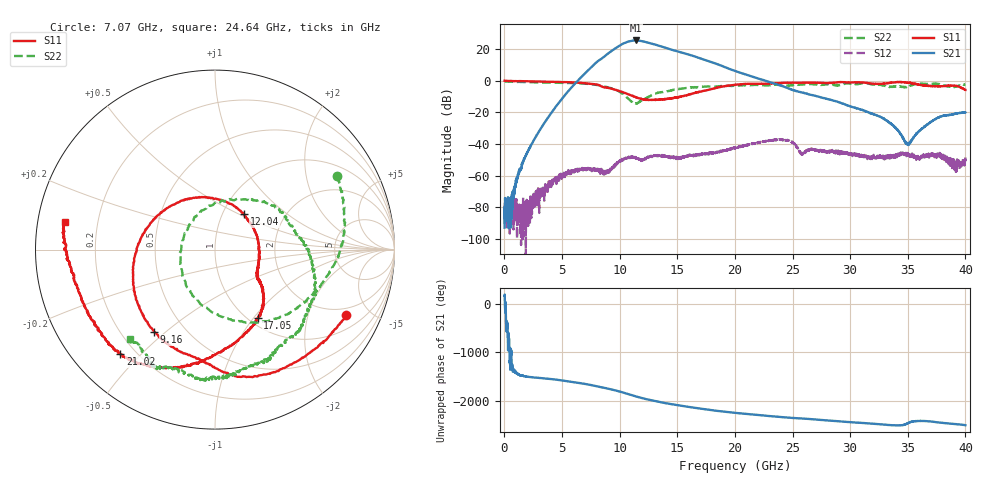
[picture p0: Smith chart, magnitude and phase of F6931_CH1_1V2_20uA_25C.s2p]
!Keysight Technologies,M9807A,MY58100526,A.15.20.05
!Date: Wednesday, October 25, 2023 15:38:21
!Correction: S11(C  2-Port  )
!S21(C  2-Port  )
!S12(C  2-Port  )
!S22(C  2-Port  )
!S2P File: Measurements: S11, S21, S12, S22:
# Hz S  dB  R 50
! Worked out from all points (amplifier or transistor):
!   4000 points, 10 MHz to 40 GHz, reference 50 ohm
!   highest |S21| = 25.3 dB at 11.4 GHz (marker M1)
!   |S21| within 3 dB of that: 10.05 GHz to 13.25 GHz (3.197 GHz wide, 27.4 % of centre)
!   unconditionally stable (mu >= 1): start of sweep to end of sweep
!   at 6.67 GHz: K = 25.76, MAG = 12.1 dB, |S12| = -56.2 dB
!   at 20.01 GHz: K = 8.07, MAG = 12.3 dB, |S12| = -42.6 dB
!   at 40 GHz: K = 434.07, MAG = -15.2 dB, |S12| = -48.6 dB
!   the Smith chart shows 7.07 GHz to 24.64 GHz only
!   S11 on the Smith chart (normalised r, x): 7.07 GHz: 1.62, -3.55; 9.16 GHz: 0.34, -0.46; 12.04 GHz: 1.26, +0.53; 17.05 GHz: 1.10, -1.05; 21.02 GHz: 0.14, -0.44; 24.64 GHz: 0.08, +0.09
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1e7  -0.09 179.7  -92.96 154.5  -90.72 95.2  -0.56 179.8
6.68e9  -1.52 -12.2  2.28 168.6  -56.44 69.7  -1.85 39.5
7.07e9  -1.76 -26.6  5.15 152.7  -55.41 57.9  -1.98 31.0
8.13e9  -2.68 -74.9  12.41 102.6  -56.56 -7.3  -2.90 4.2
9.16e9  -4.89 -126.4  18.02 49.8  -55.74 -121.0  -4.67 -28.7
9.8e9  -6.22 -159.1  21.20 12.8  -51.89 175.2  -6.36 -56.3
1.041e10  -7.73 168.7  23.72 -27.4  -49.01 132.5  -9.30 -94.3
1.097e10  -9.28 133.7  25.04 -67.6  -48.65 99.1  -13.06 -144.8
1.14e10  -10.48 102.4  25.34 -98.0  -48.65 77.6  -14.56 158.2
1.204e10  -11.84 50.8  24.73 -139.7  -50.07 73.2  -12.15 93.7
1.262e10  -12.18 19.0  23.66 -172.5  -48.03 54.7  -9.86 60.5
1.334e10  -12.10 -6.4  22.14 151.5  -47.74 34.6  -7.71 35.1
1.416e10  -11.38 -27.4  20.29 116.2  -48.35 15.1  -6.80 12.0
1.528e10  -10.27 -35.9  17.89 72.8  -48.72 6.5  -5.17 -9.2
1.705e10  -6.95 -58.2  13.86 10.8  -46.96 -17.1  -3.99 -37.0
1.838e10  -4.67 -90.0  10.63 -31.6  -45.27 -31.3  -3.71 -55.3
2.001e10  -2.68 -116.9  6.03 -73.9  -42.63 -53.9  -3.30 -75.4
2.102e10  -2.11 -132.2  3.61 -97.2  -40.83 -75.2  -3.05 -87.5
2.464e10  -1.40 169.5  -5.00 -172.4  -38.08 153.3  -3.29 -133.5
2.667e10  -1.37 145.6  -9.16 155.4  -42.98 128.2  -2.35 -148.8
3.334e10  -1.54 27.8  -26.21 37.0  -47.32 -5.2  -3.80 124.5
4e10  -5.94 -138.0  -20.13 33.2  -48.57 -54.6  -2.42 4.7
